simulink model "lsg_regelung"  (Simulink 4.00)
settings: Solver=ode45  StartTime=0.0  StopTime=Tstop  MaxStep=max_step  RelTol=1e-3
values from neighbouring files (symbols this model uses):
  den = [0.02 1]    [lsg_regelung_ini.m]    (also in lsg_system_ini.m; lsg_sys_kalman_ini.m; system_ini.m; sys_kalman_ini.m)
  g = 2    [lsg_regelung_ini.m]    (also in lsg_system_ini.m; lsg_sys_kalman_ini.m; system_ini.m; sys_kalman_ini.m)
  k = place(syszreg.a,syszreg.b,polc)    [gnmbeobregl_i.m]    (also in gnmbeobregs_i.m; gnmbeobreg_i.m = [ 0 0 0 ])
  Kv = -1/(C*inv(A-B*k)*B)    [lsg_regelung_ini.m]
  num = 2    [lsg_regelung_ini.m]    (also in lsg_system_ini.m; lsg_sys_kalman_ini.m; system_ini.m; sys_kalman_ini.m)
  p = [-2 -3+10*i -3-10*i]    [lsg_regelung_ini.m]    (also in lsg_system_ini.m; lsg_sys_kalman_ini.m; system_ini.m; sys_kalman_ini.m)
  Q = 1e-3    (= 0.001)    [lsg_regelung_ini.m]    (also in lsg_sys_kalman_ini.m; sys_kalman_ini.m = 1e-06)
  R = 1e-3    (= 0.001)    [lsg_regelung_ini.m]    (also in lsg_sys_kalman_ini.m; sys_kalman_ini.m = 1e-06)
  verst = 100    [lsg_regelung_ini.m]    (also in lsg_system_ini.m; lsg_sys_kalman_ini.m; system_ini.m; sys_kalman_ini.m)
  z = [1 1]    [lsg_regelung_ini.m]    (also in lsg_system_ini.m; lsg_sys_kalman_ini.m; system_ini.m; sys_kalman_ini.m)
undefined symbols (not defined in the file or in its folder): kest
libraries: simulink3 x1

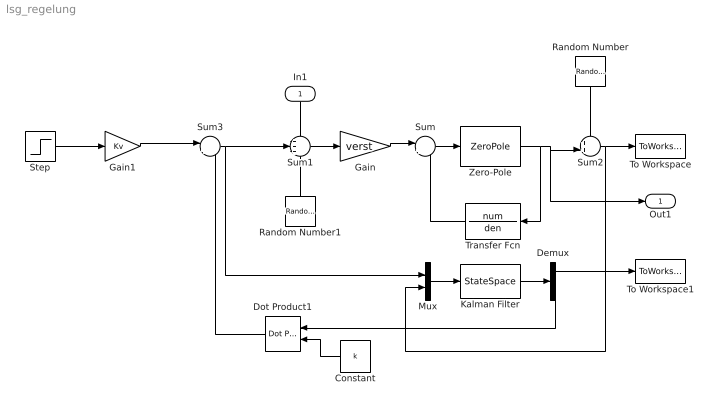
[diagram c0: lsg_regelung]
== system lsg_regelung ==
  In1 : Inport  Orientation=down  Port=1
  Constant : Constant  Orientation=left  Value=k
  Demux : Demux  Outputs=[1 4]  BusSelectionMode=off
  Dot Product1 : simulink3/Math/Dot Product  Orientation=left
  Gain : Gain  Gain=verst  Multiplication=Element-wise(K.*u)  SaturateOnIntegerOverflow=on
  Gain1 : Gain  Gain=Kv  Multiplication=Element-wise(K.*u)  SaturateOnIntegerOverflow=on
  Kalman Filter : StateSpace  A=kest.a  B=kest.b  C=kest.c  D=kest.d  X0=0  Realization=auto  AbsoluteTolerance=auto
  Mux : Mux  Inputs=2
  Random Number : RandomNumber  Orientation=down  Mean=0  Variance=R  Seed=0  SampleTime=0
  Random Number1 : RandomNumber  Orientation=up  Mean=0  Variance=Q  Seed=0  SampleTime=0
  Step : Step  Time=0  Before=0  After=100  SampleTime=0
  Sum : Sum  Inputs=|++  SaturateOnIntegerOverflow=on
  Sum1 : Sum  Inputs=+++  SaturateOnIntegerOverflow=on
  Sum2 : Sum  Inputs=++|  SaturateOnIntegerOverflow=on
  Sum3 : Sum  Inputs=|+-  SaturateOnIntegerOverflow=on
  To Workspace : ToWorkspace  VariableName=y  SampleTime=-1  SaveFormat=Array
  To Workspace1 : ToWorkspace  VariableName=ye  SampleTime=-1  SaveFormat=Array
  Transfer Fcn : TransferFcn  Orientation=left  Numerator=num  Denominator=den  Realization=auto  AbsoluteTolerance=auto
  Zero-Pole : ZeroPole  Zeros=z  Poles=p  Gain=g  AbsoluteTolerance=auto
  Out1 : Outport  Port=1
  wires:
  Transfer Fcn/1 -> Sum/2
  Sum/1 -> Zero-Pole/1
  Gain/1 -> Sum/1
  Zero-Pole/1 -> Transfer Fcn/1, Sum2/2, Out1/1
  Sum2/1 -> To Workspace/1, Mux/2
  In1/1 -> Sum1/1
  Sum1/1 -> Gain/1
  Mux/1 -> Kalman Filter/1
  Kalman Filter/1 -> Demux/1
  Demux/1 -> To Workspace1/1
  Demux/2 -> Dot Product1/1
  Constant/1 -> Dot Product1/2
  Sum3/1 -> Sum1/2, Mux/1
  Dot Product1/1 -> Sum3/2
  Step/1 -> Gain1/1
  Gain1/1 -> Sum3/1
  Random Number1/1 -> Sum1/3
  Random Number/1 -> Sum2/1
